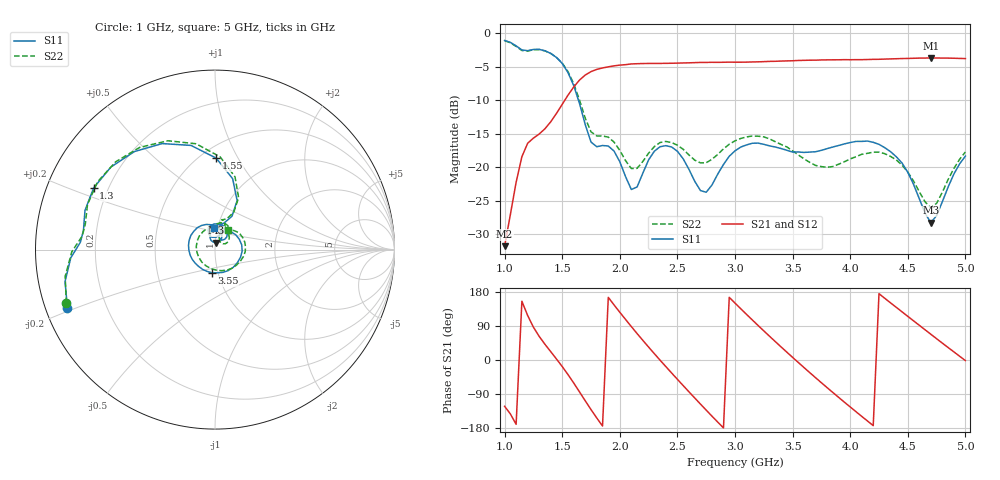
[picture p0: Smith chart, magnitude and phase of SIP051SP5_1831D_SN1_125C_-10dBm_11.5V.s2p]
# GHz  S  dB  R  50
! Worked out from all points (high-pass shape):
!   81 points, 1 GHz to 5 GHz, reference 50 ohm
!   highest |S21| = -3.69 dB at 4.7 GHz (marker M1); lowest = -31.8 dB at 1 GHz (marker M2)
!   |S21| within 3 dB of the highest: 1.67 GHz to end of sweep
!   lowest |S11| = -28.2 dB at 4.7 GHz (marker M3), VSWR 1.08, Z = 50.3 + j3.87 ohm
!   |S11| at or under -10 dB: 1.641 GHz to end of sweep
!   |S22| runs from -26.0 to -1.1 dB; largest |S21 - S12| = 0.0018
!   S11 on the Smith chart (normalised r, x): 1 GHz: 0.06, -0.19; 1.3 GHz: 0.15, +0.24; 1.55 GHz: 0.59, +0.82; 3.55 GHz: 0.93, -0.24; 5 GHz: 0.96, +0.24
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1  -1.08 -158.6  -31.75 -122.2  -31.77 -123.1  -1.11 -160.2
1.15  -2.49 176.8  -18.41 155.1  -18.38 155.1  -2.57 174.2
1.3  -2.40 153.0  -15.03 62.4  -15.01 62.5  -2.44 150.0
1.55  -5.86 89.2  -9.24 -38.4  -9.24 -38.3  -5.72 86.8
1.7  -13.62 63.0  -6.23 -107.6  -6.22 -107.7  -12.66 63.3
1.85  -16.74 85.3  -5.18 -174.3  -5.17 -174.3  -15.32 77.2
2.05  -21.39 73.1  -4.68 107.0  -4.67 107.0  -19.00 66.9
2.2  -20.86 111.8  -4.52 51.8  -4.52 51.9  -19.12 90.4
2.35  -16.92 93.2  -4.50 -0.6  -4.50 -0.6  -16.29 79.0
2.5  -17.60 62.1  -4.46 -51.0  -4.45 -51.0  -16.69 57.2
2.65  -22.06 46.6  -4.38 -100.1  -4.37 -100.1  -18.92 49.5
2.85  -21.01 72.2  -4.34 -163.8  -4.33 -163.9  -18.07 55.2
3  -17.54 47.3  -4.32 150.2  -4.31 150.2  -16.05 39.1
3.25  -16.57 -16.3  -4.24 76.8  -4.23 76.9  -15.46 -4.1
3.55  -17.71 -98.2  -4.06 -6.7  -4.06 -6.7  -18.15 -71.6
3.7  -17.67 -134.7  -4.02 -46.9  -4.01 -46.9  -19.71 -118.8
3.95  -16.50 170.6  -3.94 -111.4  -3.94 -111.4  -19.16 154.6
4.15  -16.08 128.7  -3.92 -160.9  -3.92 -160.9  -17.91 98.9
4.35  -17.66 89.2  -3.83 150.8  -3.83 150.8  -18.37 56.7
4.55  -22.54 59.9  -3.73 103.3  -3.73 103.3  -22.04 30.1
4.7  -28.25 83.4  -3.69 67.9  -3.68 68.0  -26.02 47.9
5  -18.32 93.5  -3.78 -1.5  -3.78 -1.5  -17.70 57.6
